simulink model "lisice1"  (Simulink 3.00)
settings: Solver=ode45  StartTime=0.0  StopTime=10  MaxStep=0.1  RelTol=1e-3  AbsTol=1e-3
libraries: simulink3 x1

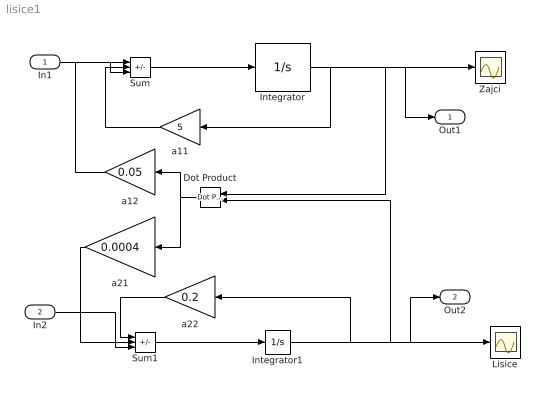
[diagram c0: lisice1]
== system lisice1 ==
  In1 : Inport  Port=1  PortWidth=-1  SampleTime=-1  DataType=auto
  In2 : Inport  Port=2  PortWidth=-1  SampleTime=-1  DataType=auto
  Dot Product : simulink3/Math/Dot Product  Orientation=left
  Integrator : Integrator  ExternalReset=none  InitialConditionSource=internal  InitialCondition=520  LimitOutput=off  UpperSaturationLimit=inf  LowerSaturationLimit=-inf  ShowSaturationPort=off  ShowStatePort=off  AbsoluteTolerance=auto
  Integrator1 : Integrator  ExternalReset=none  InitialConditionSource=internal  InitialCondition=85  LimitOutput=off  UpperSaturationLimit=inf  LowerSaturationLimit=-inf  ShowSaturationPort=off  ShowStatePort=off  AbsoluteTolerance=auto
  Lisice : Scope
  Sum : Sum  Inputs=-++  SaturateOnIntegerOverflow=on
  Sum1 : Sum  Inputs=-++  SaturateOnIntegerOverflow=on
  Zajci : Scope
  a11 : Gain  Orientation=left  Gain=5  SaturateOnIntegerOverflow=on
  a12 : Gain  Orientation=left  Gain=0.05  SaturateOnIntegerOverflow=on
  a21 : Gain  Orientation=left  Gain=0.0004  SaturateOnIntegerOverflow=on
  a22 : Gain  Orientation=left  Gain=0.2  SaturateOnIntegerOverflow=on
  Out1 : Outport  Port=1
  Out2 : Outport  Port=2
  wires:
  Sum/1 -> Integrator/1
  Sum1/1 -> Integrator1/1
  Integrator/1 -> a11/1, Dot Product/1, Zajci/1, Out1/1
  Integrator1/1 -> a22/1, Dot Product/2, Lisice/1, Out2/1
  a22/1 -> Sum1/1
  a11/1 -> Sum/2
  a12/1 -> Sum/1
  Dot Product/1 -> a12/1, a21/1
  a21/1 -> Sum1/2
  In1/1 -> Sum/3
  In2/1 -> Sum1/3
